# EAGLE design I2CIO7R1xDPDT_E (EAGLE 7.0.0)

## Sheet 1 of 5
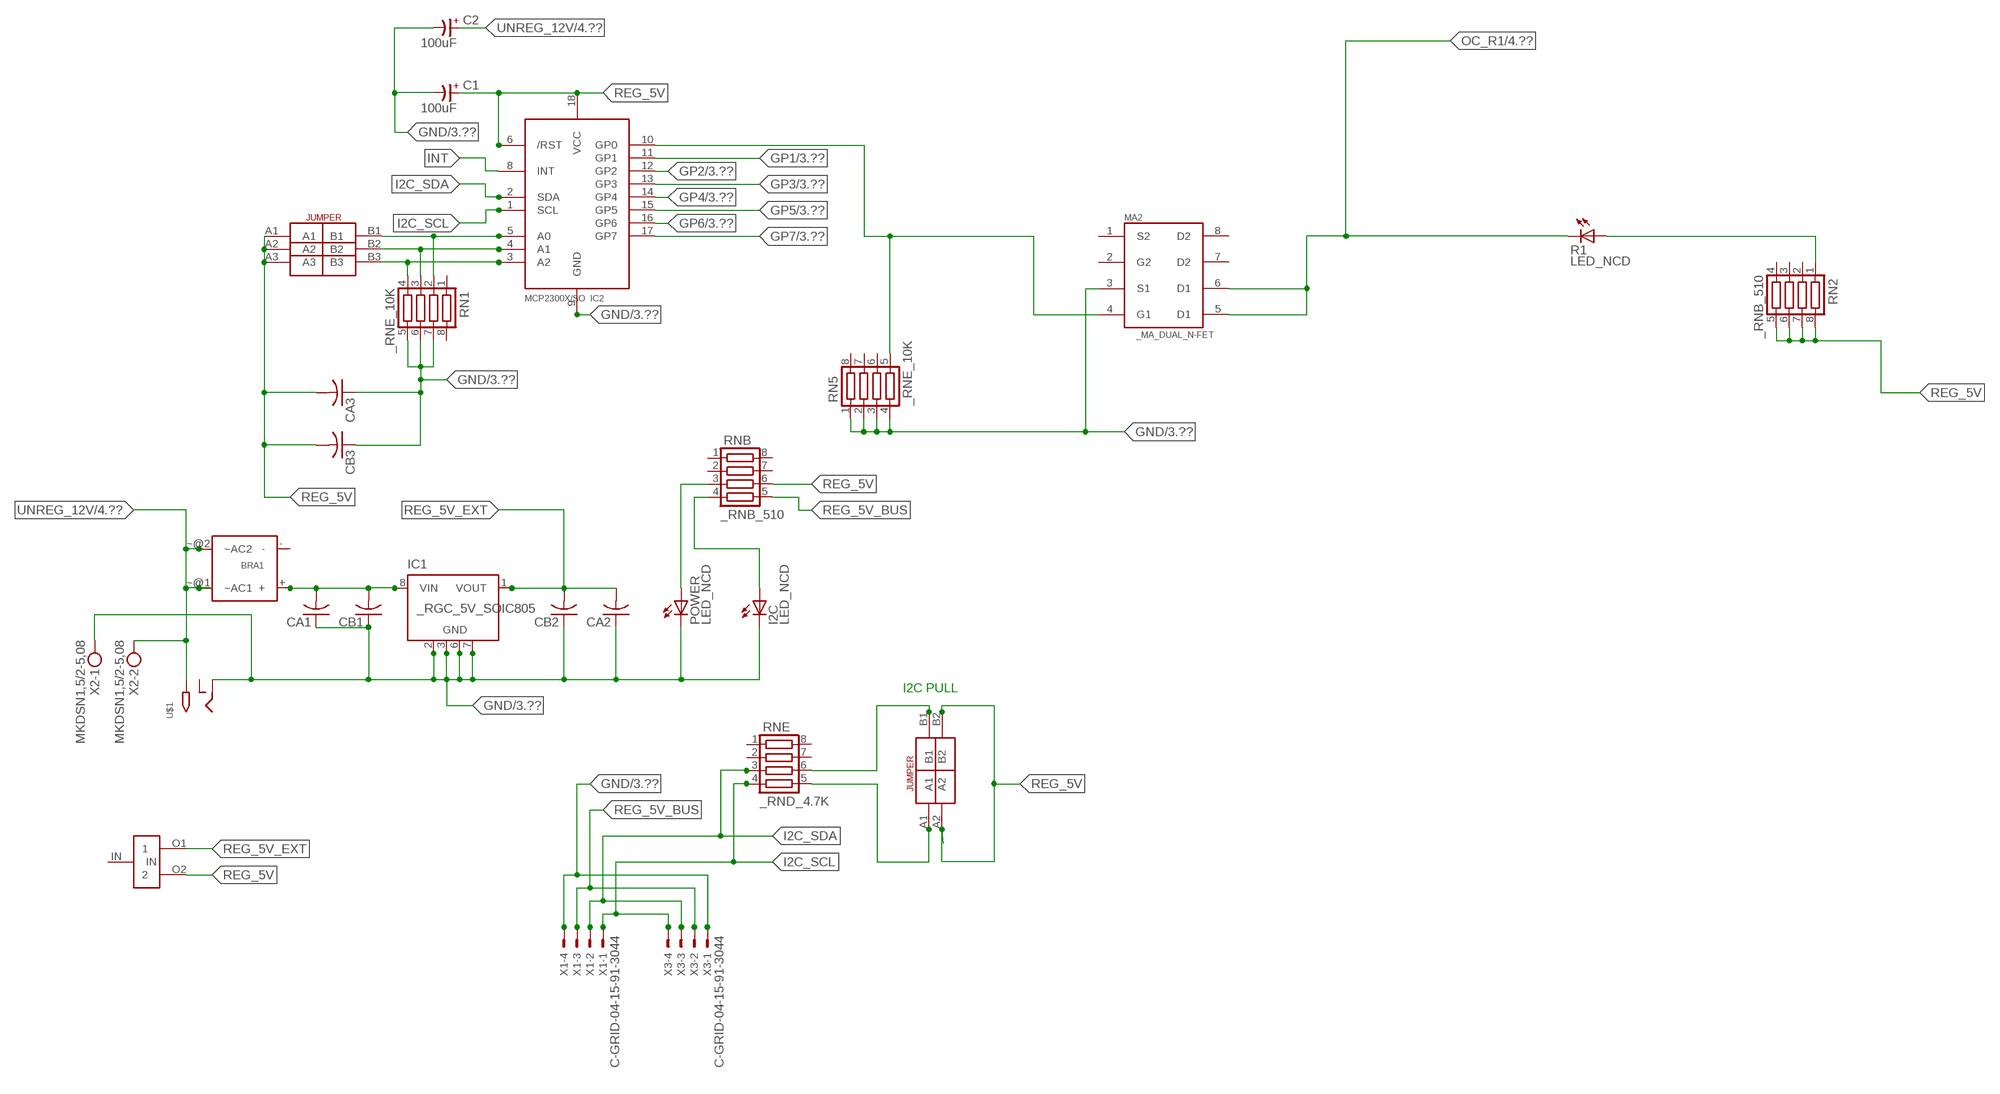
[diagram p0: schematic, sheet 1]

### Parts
BRA1  MB2S_  [MB2S]
C1  100uF  CP-E-025X060  [E-025X060]
C2  100uF  CP-E-025X060  [E-025X060]
CA1  CC1206KRX7R9BB104C1206K  [CC1206KRX7R9BB104]
CA2  CC1206KRX7R9BB104C1206K  [CC1206KRX7R9BB104]
CA3  CC1206KRX7R9BB104C1206K  [CC1206KRX7R9BB104]
CB1  TMK316F106ZL-TC1206K  [TMK316F106ZL-T]
CB2  TMK316F106ZL-TC1206K  [TMK316F106ZL-T]
CB3  TMK316F106ZL-TC1206K  [TMK316F106ZL-T]
I2C  LED_NCD  [CHIPLED_0603]
IC1  _RGC_5V_SOIC805  [_RGC_5V_SOIC8]
IC2  MCP2300X/SO  [SO18W]
MA2  _MA_DUAL_N-FET  [_MA_DUAL_N-FET]
POWER  LED_NCD  [CHIPLED_0603]
R1  LED_NCD  [CHIPLED_0603]
RN1  _RNE_10K  [RNE]
RN2  _RNB_510  [RNB]
RN5  _RNE_10K  [RNE]
RNB  _RNB_510  [RNB]
RNE  _RND_4.7K  [RND]
U$1  2.1MMJACK  [PJ-102A]
U$3  JUMPER_2X2  [JUMPER_2X2]
U$5  LINK_2  [LINK_2]
U$18  JUMPER_3X2  [JUMPER_3X2]
X1  C-GRID-04-15-91-3044  [15-91-04]
X2  MKDSN1,5/2-5,08  [MKDSN1,5/2-5,08]
X3  C-GRID-04-15-91-3044  [15-91-04]

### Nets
GND: C1.- C2.- CA1.1 CA2.1 CA3.1 CB1.1 CB2.1 CB3.1 I2C.C IC1.2(GND) IC1.3(GND) IC1.6(GND) IC1.7(GND) IC2.9(GND) MA2.3(S1) POWER.C RN1.5 RN1.6 RN1.7 RN5.1 RN5.2 RN5.3 RN5.4 U$1.RING X1.4 X2.1 X3.1 ; also sheet 3
GP1: IC2.11(GP1) ; also sheet 3
GP2: IC2.12(GP2) ; also sheet 3
GP3: IC2.13(GP3) ; also sheet 3
GP4: IC2.14(GP4) ; also sheet 3
GP5: IC2.15(GP5) ; also sheet 3
GP6: IC2.16(GP6) ; also sheet 3
GP7: IC2.17(GP7) ; also sheet 3
I2C_SCL: IC2.1(SCL) RNE.4 X1.1 X3.4
I2C_SDA: IC2.2(SDA) RNE.3 X1.2 X3.3
INT: IC2.8(INT)
N$1: BRA1.+ CA1.2 CB1.2 IC1.8(VIN)
N$2: POWER.A RNB.3
N$3: I2C.A RNB.4
N$4: RNE.5 U$3.A1
N$5: RNE.6 U$3.B1
N$6: IC2.5(A0) RN1.2 U$18.B1
N$7: IC2.4(A1) RN1.3 U$18.B2
N$8: IC2.3(A2) RN1.4 U$18.B3
N$23: IC2.10(GP0) MA2.4(G1) RN5.5
N$32: R1.A RN2.1
OC_R1: MA2.5(D1) MA2.6(D1) R1.C ; also sheet 4
REG_5V: C1.+ CA3.2 CB3.2 IC2.6(/RST) IC2.18(VCC) RN2.5 RN2.6 RN2.7 RN2.8 RNB.6 U$3.A2 U$3.B2 U$5.O2 U$18.A1 U$18.A2 U$18.A3
REG_5V_BUS: RNB.5 X1.3 X3.2
REG_5V_EXT: CA2.2 CB2.2 IC1.1(VOUT) U$5.O1
UNREG_12V: BRA1.~@1(~AC1) BRA1.~@2(~AC2) C2.+ U$1.TIP X2.2 ; also sheet 4
Unconnected: BRA1.- IC1.4(NC) IC1.5(NC) MA2.2(G2) MA2.7(D2) MA2.8(D2) RN1.1 RN1.8 RN2.2 RN2.3 RN2.4 RN5.6 RN5.7 RN5.8 RNB.1 RNB.2 RNB.7 RNB.8 RNE.1 RNE.2 RNE.7 RNE.8 U$1.RING_SW U$5.IN

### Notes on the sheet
- I2C PULL

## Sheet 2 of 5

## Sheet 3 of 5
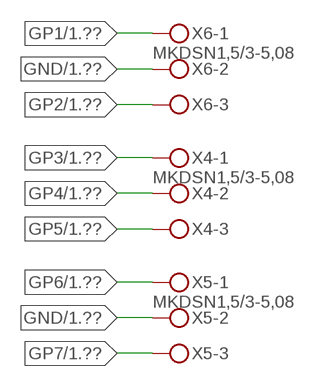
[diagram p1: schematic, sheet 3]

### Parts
X4  MKDSN1,5/3-5,08  [MKDSN1,5/3-5,08]
X5  MKDSN1,5/3-5,08  [MKDSN1,5/3-5,08]
X6  MKDSN1,5/3-5,08  [MKDSN1,5/3-5,08]

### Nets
GND: X5.2 X6.2 ; also sheet 1
GP1: X6.1 ; also sheet 1
GP2: X6.3 ; also sheet 1
GP3: X4.1 ; also sheet 1
GP4: X4.2 ; also sheet 1
GP5: X4.3 ; also sheet 1
GP6: X5.1 ; also sheet 1
GP7: X5.3 ; also sheet 1

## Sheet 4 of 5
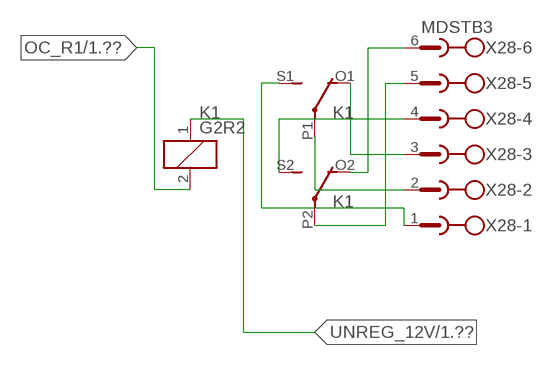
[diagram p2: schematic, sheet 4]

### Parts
K1  G2R2  [G2R2]
X28  MDSTB3  [MDSTB3]

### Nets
N$203: K1.P2(3:COM) X28.5
N$204: K1.O2(3:NC) X28.6
N$205: K1.S2(3:NO) X28.4
N$206: K1.P1(2:COM) X28.2
N$207: K1.O1(2:NC) X28.3
N$208: K1.S1(2:NO) X28.1
OC_R1: K1.2(1:C2) ; also sheet 1
UNREG_12V: K1.1(1:C1) ; also sheet 1

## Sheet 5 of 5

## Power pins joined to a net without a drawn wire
S2: MA2.1(S2)

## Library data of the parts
BRA1 = NCD_ULTIMATE_LIBRARY:MB2S: Bridge Rectifier BRA MB2S 200V 500ma Digikey MB2S-TPMSTR-ND/MB2S-TP
C1 C2 = NCD_ULTIMATE_LIBRARY:CP-: Capacitors All Kinds POLARIZED CAP
CA1-CA3 = NCD_ULTIMATE_LIBRARY:CC1206KRX7R9BB104: Capacitor CA .1uF 50V SMT C1206K CC1206KRX7R9BB104
CB1-CB3 = NCD_ULTIMATE_LIBRARY:TMK316F106ZL-T: Capacitor CB 10uF SMT 1206 TMK316F106ZL-T
I2C POWER = NCD_ULTIMATE_bhaskar:LED_NCD
IC1 = NCD_ULTIMATE_LIBRARY:_RGC_5V_SOIC8: Regulator Linear 5V Chip Positive VOLTAGE REGULATOR Digikey 497-7267-2-ND/L78L05CD13TR
IC2 = NCD_ULTIMATE_LIBRARY:MCP2300X: Semiconductor Port Expander I/O 8-Bit I2C MCP23008 Inexpensive i2c i/o expander - 8 general purpose i/o pins with optional pullups
K1 = NCD_ULTIMATE_LIBRARY:G2R2: RELAY 2 x switch, Omron
MA2 = NCD_ULTIMATE_LIBRARY:_MA_DUAL_N-FET: FET Dual N-Channel 8-SOIC NMOSFET Digikey 785-1064-2-ND/AO4842
R1 = NCD_ULTIMATE_LIBRARY:LED_NCD: LED Digikey 754-1132-2-ND/APT2012SRCPRV
RN1 RN5 = NCD_ULTIMATE_LIBRARY:_RNE_10K: Resistor Array RNE SMT 10K x 4 Single Resistor Source: http://www.ctscorp.com/components/Datasheets/CTSChipArrayDs.pdf Digikey 742C083103JPTR-ND/742C083103JP; OC_FARNELL: unknown; OC_NEWARK: unknown
RN2 RNB = NCD_ULTIMATE_LIBRARY:_RNB_510: Resistor Array RNB SMT 510 x 4 Single Resistor Source: http://www.ctscorp.com/components/Datasheets/CTSChipArrayDs.pdf Digikey 742C083511JPTR-ND/ 742C083511JP; OC_FARNELL: unknown; OC_NEWARK: unknown
RNE = NCD_ULTIMATE_LIBRARY:_RND_4.7K: Resistor Array RND SMT 4.7K x 4 Single Resistor Source: http://www.ctscorp.com/components/Datasheets/CTSChipArrayDs.pdf Digikey 742C083472JPTR-ND/742C083472JP; OC_FARNELL: unknown; OC_NEWARK: unknown
U$1 = NCD_ULTIMATE_CONNECTORS:2.1MMJACK: 2.1mm x 5.5mm DC jack with internal switch. Digikey part #PJ-102A, 4UCON part #05537 By microbuilder.eu
U$3 = NCD_ULTIMATE_CONNECTORS:JUMPER_2X2
U$5 = NCD_ULTIMATE_LIBRARY:LINK_2: PAD_top
U$18 = NCD_ULTIMATE_CONNECTORS:JUMPER_3X2
X1 X3 = NCD_ULTIMATE_CONNECTORS:C-GRID-04: CONNECTOR 4-Pos I2C wire to board 2.54 mm (0.100") pitch header Digikey WM1342-ND/0015912045; OC_FARNELL: unknown; OC_NEWARK: unknown
X2 = NCD_ULTIMATE_CONNECTORS:MKDSN1,5/2-5,08: MKDSN 1,5/ 2-5,08 Printklemme
X4-X6 = NCD_ULTIMATE_CONNECTORS:MKDSN1,5/3-5,08: MKDSN 1,5/ 3-5,08 Printklemme Nennstrom: 13,5 A Nennspannung: 250 V Rastermaß: 5,08 mm Polzahl: 3 Anschlussart: Schraubanschluss Montage: Löten Anschlussrichtung Leiter/Platine: 0 ° Artikelnummer: 1729131 Source: http://eshop.phoenixcontact.com .. 1729131.pdf
X28 = NCD_ULTIMATE_LIBRARY:MDSTB3: PHOENIX

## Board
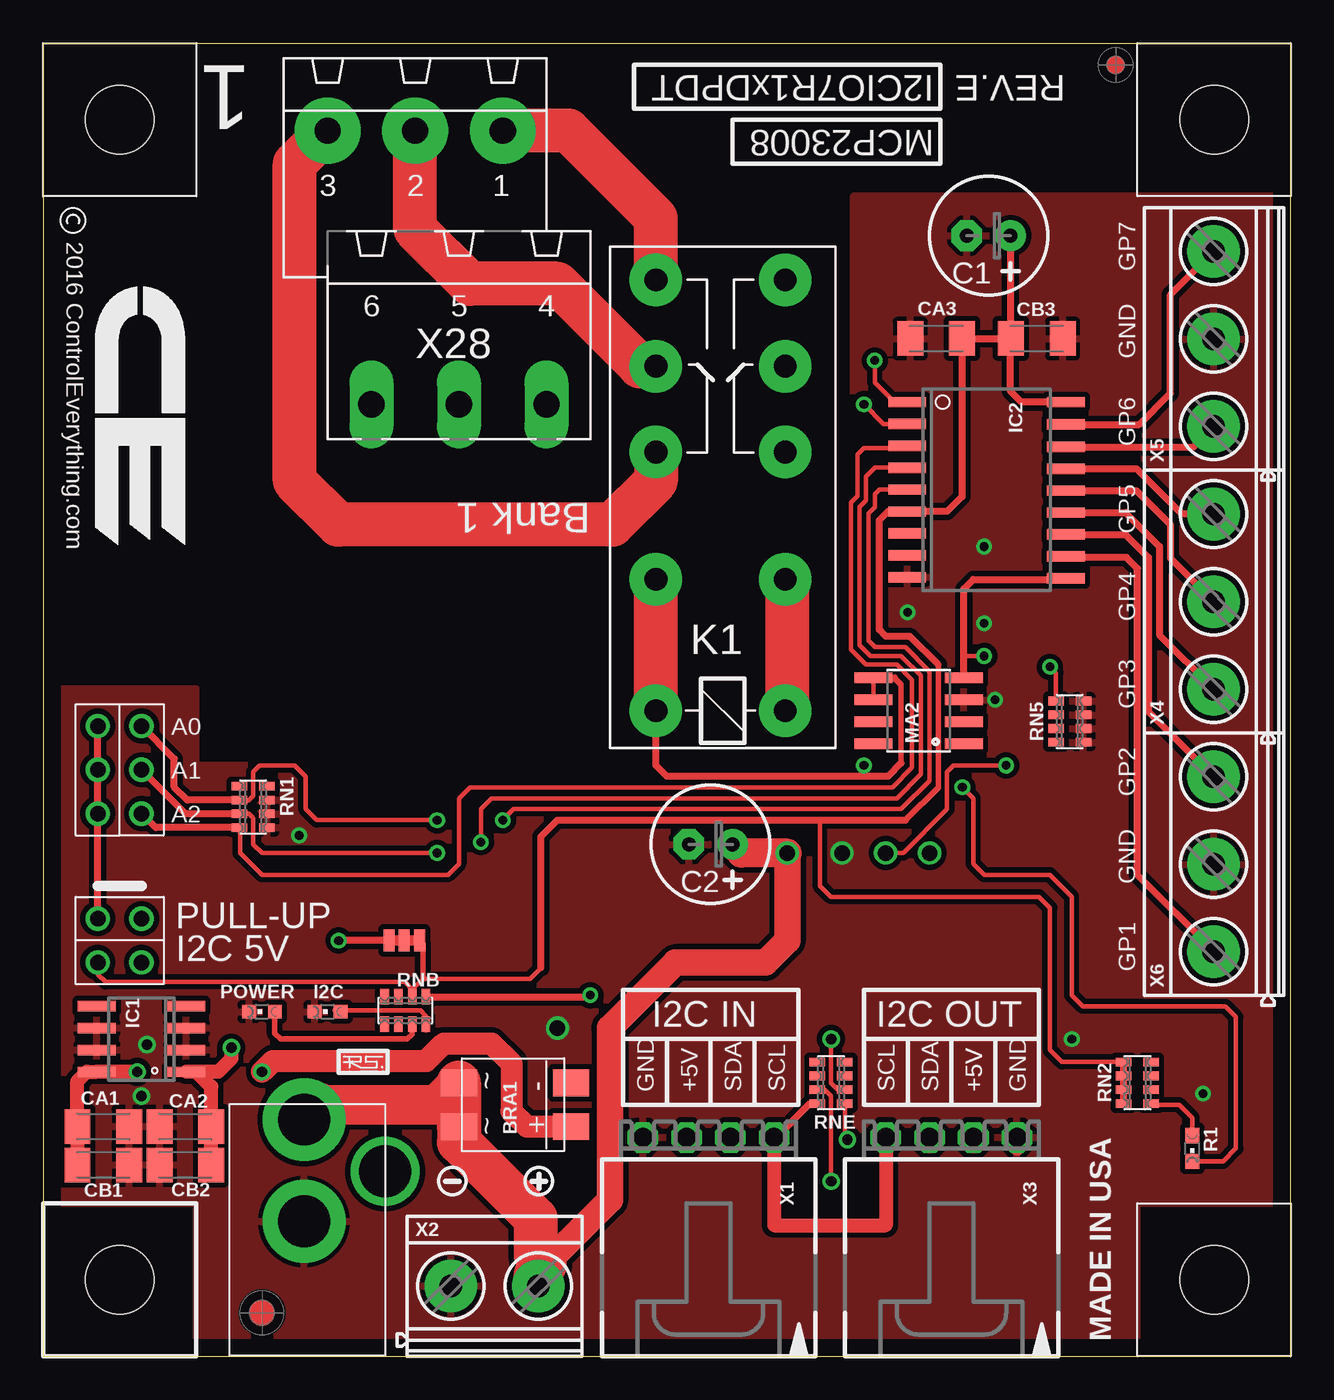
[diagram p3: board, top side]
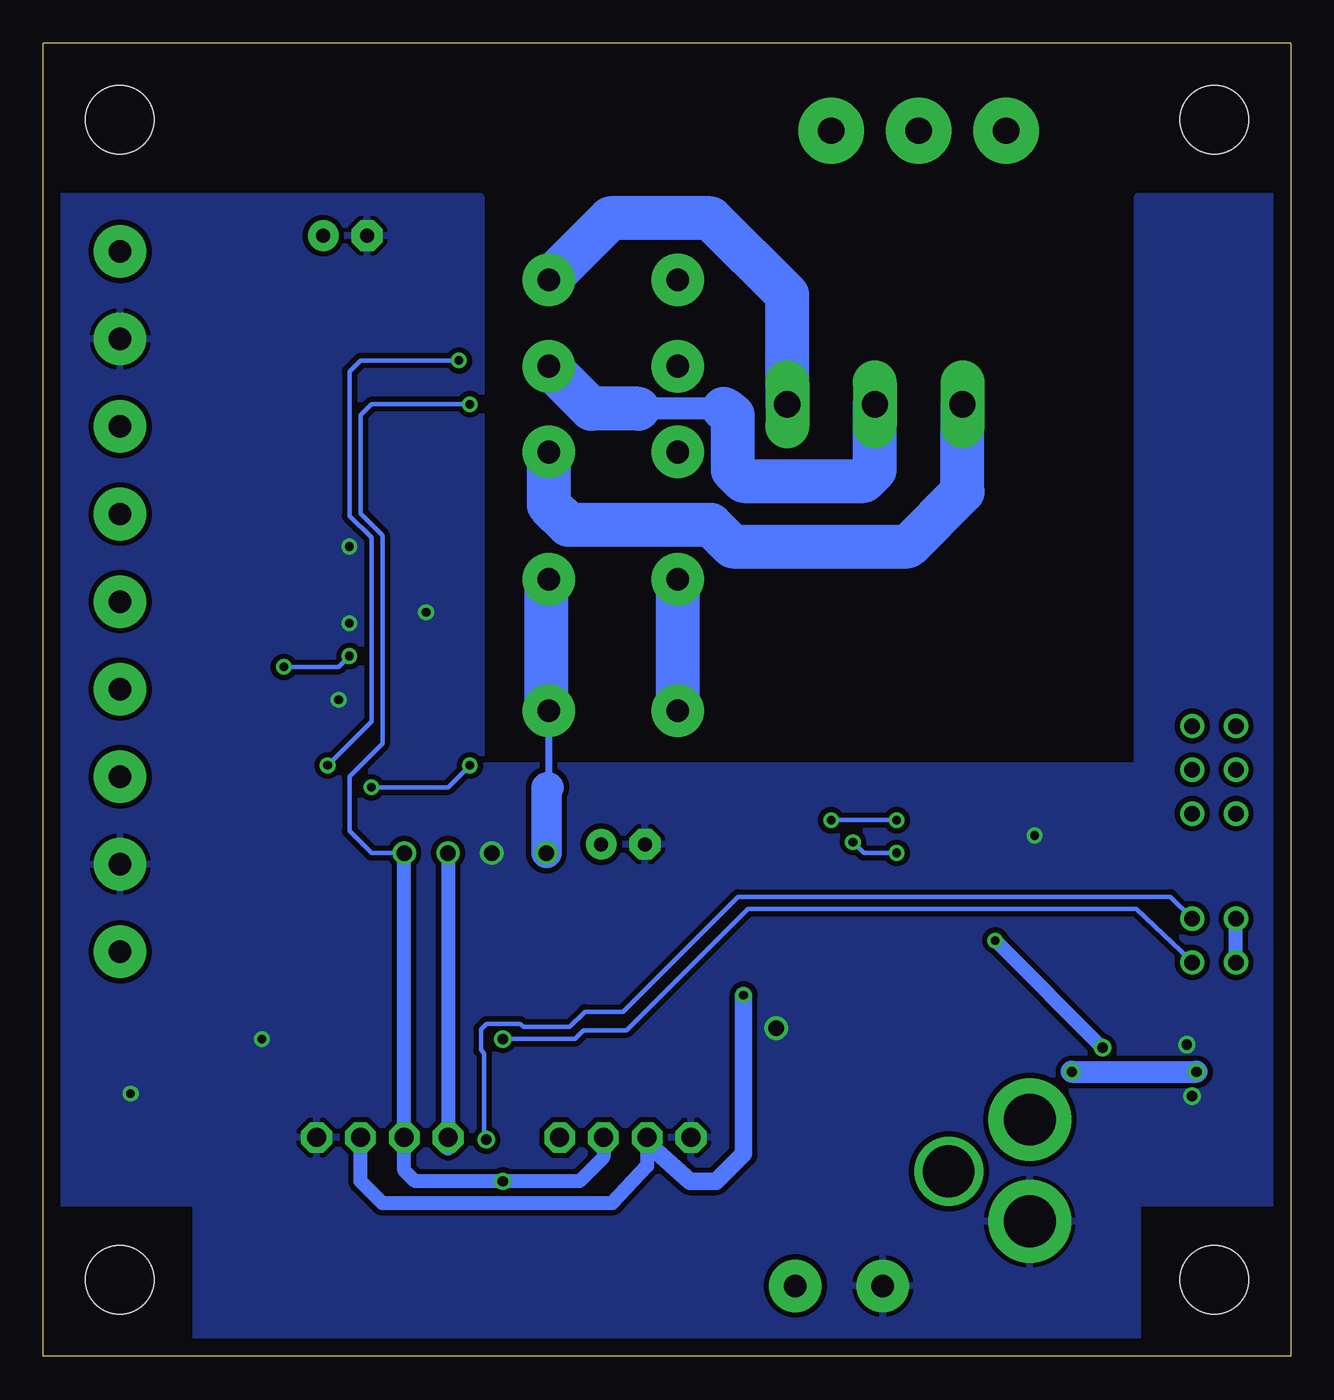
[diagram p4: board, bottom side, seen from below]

Size 72.39 x 76.2 mm. Coordinates in mm from the lower left corner, seen from the top.
Outline: 59.69,0 0,0 0,76.2 72.39,76.2 72.39,0 59.69,0
Outline: 59.69,0 61.58,0
Copper layers (1*16): Top 0.035mm / dielectric 1.5mm / Bottom 0.035mm
Design rules "default": minimum track width 10mil, minimum drill 24mil, track to track 8mil, track to pad 8mil, pad to pad 8mil, via to via 8mil, smd to smd 8mil, copper to edge 40mil, drill to drill 8mil, minimum pad ring 10mil, minimum via ring 8mil, stop-mask expansion 4mil, vias tented up to drill 0mil, thermal gap 10mil
Holes 3.96 mm at 4.45,4.45

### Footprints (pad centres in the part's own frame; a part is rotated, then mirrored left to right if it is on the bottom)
MB2S = smd 1.55 x 2.1: + 0,-6.5; - 2.54,-6.5; ~@1 0,0; ~@2 2.54,0
E-025X060 = drill 0.813 pad 1.778: + -1.27,0 | drill 0.813 pad 1.778 octagon: - 1.27,0
CC1206KRX7R9BB104 = smd 1.5 x 2: 1 -1.5,0; 2 1.5,0
TMK316F106ZL-T = smd 1.5 x 2: 1 -1.5,0; 2 1.5,0
CHIPLED_0603 = smd 0.8 x 0.8: A 0,-0.75; C 0,0.75
_RGC_5V_SOIC8 = smd 0.6 x 2.2: 1 -1.905,-2.6; 2 -0.635,-2.6; 3 0.635,-2.6; 4 1.905,-2.6; 5 1.905,2.6; 6 0.635,2.6; 7 -0.635,2.6; 8 -1.905,2.6
SO18W = smd 0.6 x 2.2: 1 -4.445,-4.6; 2 -3.175,-4.6; 3 -1.905,-4.6; 4 -0.635,-4.6; 5 0.635,-4.6; 6 1.905,-4.6; 7 3.175,-4.6; 8 4.445,-4.6; 9 5.715,-4.6; 10 5.775,4.6; 11 4.505,4.6; 12 3.235,4.6; 13 1.965,4.6; 14 0.695,4.6; 15 -0.575,4.6; 16 -1.845,4.6; 17 -3.145,4.6; 18 -4.445,4.6
G2R2 = drill 1.321 pad 3.048: 1 -2.54,-3.683; 2 -2.54,3.81; 3 5.08,-3.683; 4 5.08,3.81; O1 12.471,3.81; O2 12.471,-3.683; P1 17.45,3.81; P2 17.45,-3.683; S1 22.454,3.81; S2 22.454,-3.683
_MA_DUAL_N-FET = smd 0.61 x 2.21: 1 -1.905,-2.616; 2 -0.635,-2.616; 3 0.635,-2.616; 4 1.905,-2.616; 5 1.905,2.616; 6 0.635,2.616; 7 -0.635,2.616; 8 -1.905,2.616
CHIPLED_0603' = smd 0.8 x 0.876: A 0,-0.75; C 0,0.75
RNE = smd 0.5 x 0.9: 1 -1.2,-0.8; 2 -0.4,-0.8; 3 0.4,-0.8; 4 1.2,-0.8; 5 1.2,0.8; 6 0.4,0.8; 7 -0.4,0.8; 8 -1.2,0.8
RNB = smd 0.5 x 0.9: 1 -1.2,-0.8; 2 -0.4,-0.8; 3 0.4,-0.8; 4 1.2,-0.8; 5 1.2,0.8; 6 0.4,0.8; 7 -0.4,0.8; 8 -1.2,0.8
RND = smd 0.5 x 0.9: 1 -1.2,-0.8; 2 -0.4,-0.8; 3 0.4,-0.8; 4 1.2,-0.8; 5 1.2,0.8; 6 0.4,0.8; 7 -0.4,0.8; 8 -1.2,0.8
PJ-102A = drill 3 pad 4.8: RING 0.1,-3.39; TIP 0.1,-9.29 | drill 3 pad 3.251: RING_SW -4.6,-6.29
JUMPER_2X2 = drill 0.9: A1 0,2.54; A2 0,0; B1 2.54,2.54; B2 2.54,0
PCB_MOUNTING_HOLE = hole 3.962: 4.445,4.445
LINK_2 = smd 1.27 x 0.635: IN 0,0; O1 0,0.889; O2 0,-0.889
JUMPER_3X2 = drill 0.9: A1 0,5.08; A2 0,2.54; A3 0,0; B1 2.54,5.08; B2 2.54,2.54; B3 2.54,0
15-91-04 = drill 1.1 pad 1.778 octagon: 1 -3.81,-7.62; 2 -1.27,-7.62; 3 1.27,-7.62; 4 3.81,-7.62
MKDSN1,5/2-5,08 = drill 1.3 pad 3.048: 1 -2.561,0.025; 2 2.519,0.025
MKDSN1,5/3-5,08 = drill 1.3 pad 3.048: 1 -7.641,0.025; 2 -2.561,0.025; 3 2.519,0.025
MDSTB3 = drill 1.524 pad 3.81: 1 -3.81,-10.795; 2 1.27,-10.795; 3 6.35,-10.795 | drill 1.524 pad 2.54 long: 4 -6.35,5.08; 5 -1.27,5.08; 6 3.81,5.08

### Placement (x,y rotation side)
BRA1  24.13,13.34 90 top
C1  54.86,65.02 180 top
C2  38.73,29.72 180 top
CA1  3.49,13.34 180 top
CA2  8.26,13.34 0 top
CA3  51.82,59.05 0 top
CB1  3.49,11.11 180 top
CB2  8.26,11.11 0 top
CB3  57.66,59.05 180 top
I2C  16.51,20 90 top
IC1  5.71,18.41 90 top
IC2  54.74,50.93 270 top
K1  39.37,40.01 90 top
MA2  50.8,37.47 90 top
POWER  12.7,20 90 top
R1  LED_NCD  [CHIPLED_0603']  66.67,12.06 180 top
RN1  12.19,31.88 270 top
RN2  63.5,15.88 90 top
RN5  59.56,36.83 90 top
RNB  21.02,20.07 0 top
RNE  45.72,15.88 270 top
U$1  15.24,4.45 180 top
U$3  3.17,25.4 270 top
U$4  PCB_MOUNTING_HOLE  [PCB_MOUNTING_HOLE]  72.39,67.31 90 top
U$5  20.95,24.13 90 top
U$6  PCB_MOUNTING_HOLE  [PCB_MOUNTING_HOLE]  72.39,0 90 top
U$7  PCB_MOUNTING_HOLE  [PCB_MOUNTING_HOLE]  8.89,67.31 90 top
U$10  [VISION_REF15]  12.7,2.54 0 top
U$18  3.17,31.5 0 top
U$19  [VISION_REF10]  62.23,74.93 0 top
U$21  [ICON_USA]  61.98,0.89 90 top
U$22  [ICON_MINUS]  23.75,10.16 180 top
U$24  [ICON_PLUS]  28.77,10.16 90 top
X1  38.61,5.08 180 top
X2  26.23,4.06 0 top
X3  52.7,5.08 180 top
X4  67.94,46.35 90 top
X5  67.94,61.59 90 top
X6  67.94,31.11 90 top
X28  22.86,60.33 180 top

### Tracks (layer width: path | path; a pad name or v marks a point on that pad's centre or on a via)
GND  (via drill 0.5, 0.6, 0.9)
  Top 0.406: 34.8,12.38 X1.4
  Top 0.813: X3.1 56.52,12.06
  other vias: 5.71,15.11 6.03,18.1 46.35,29.21 29.84,19.05 14.86,30.23 54.61,42.55 54.61,46.99 59.69,18.41 67.31,15.24 50.16,43.18 55.24,38.1
  pour Bottom (isolate 0.305): -0.64,8.89 8.89,8.89 8.89,0 63.5,0 63.5,8.89 71.75,8.89 71.75,67.31 46.99,67.31 46.99,34.29 8.89,34.29 8.89,67.31 -0.64,67.31
  pour Top (isolate 0.305): -0.64,8.89 8.89,8.89 8.89,0 63.5,0 63.5,8.89 71.75,8.89 71.75,67.31 46.99,67.31 46.99,34.29 8.89,34.29 8.89,38.73 -0.64,38.73
GP1
  Top 0.406: X6.1 67.92,23.52 63.5,27.94 63.5,45.72 62.87,46.35 59.4,46.35 IC2.11
GP2
  Top 0.406: IC2.12 62.8,47.69 64.14,46.35 64.14,37.42 X6.3
GP3
  Top 0.406: IC2.13 62.8,48.96 64.77,46.99 64.77,41.86 X4.1
GP4
  Top 0.406: IC2.14 63.43,50.23 65.41,48.26 65.41,46.31 X4.2
GP5
  Top 0.406: IC2.15 63.43,51.5 66.04,48.9 67.9,48.9 X4.3
GP6
  Top 0.406: IC2.16 66.74,52.77 X5.1
GP7
  Top 0.406: IC2.17 63.6,54.07 65.41,55.88 65.41,61.6 X5.3
I2C_SCL  (via drill 0.5, 0.9)
  Top 0.254: IC2.1 49.4,55.37 48.26,56.52 v48.26,57.78 | v55.88,34.29 52.83,34.29 52.45,33.91 52.45,31.75 49.91,29.21 v48.9,29.21
  Top 0.406: RNE.4 44.51,14.68 42.42,12.57
  Top 0.813: X3.4 48.9,7.62 42.42,7.62 42.42,12.57 X1.1
  Bottom 0.254: v48.26,57.78 53.98,57.78 54.61,57.15 54.61,48.77 53.34,47.5 53.34,36.83 v55.88,34.29
  Bottom 0.813: v48.9,29.21 X3.4 48.9,12.06
I2C_SDA  (via drill 0.5, 0.6, 0.9)
  Top 0.254: RNE.3 45.36,15.47 45.72,15.11 v45.72,10.16 | IC2.2 48.77,54.1 v47.62,55.24
  Top 0.61: X3.3 51.44,12.06 | X1.2 39.88,12.38
  Bottom 0.254: v47.62,55.24 53.34,55.24 53.98,54.61 53.98,48.9 52.7,47.62 52.7,35.56 54.61,33.66 54.61,30.48 53.34,29.21 v51.44,29.21
  Bottom 0.406: 39.88,12.38 X1.2
  Bottom 0.813: 39.88,12.38 39.88,11.56 41.27,10.16 v45.72,10.16 50.8,10.16 51.44,10.79 X3.3 v51.44,29.21
N$1  (via drill 0.6)
  Top 0.813: CB1.2 CA1.2 1.99,15.96 2.54,16.51 IC1.8 v5.46,16.51
  Top 1.27: v12.7,16.51 13.34,17.14 22.23,17.14 23.24,18.16 26.04,18.16 27.18,17.02 27.18,14.22 28.07,13.34 BRA1.+
  Bottom 1.27: v12.7,16.51 v5.46,16.51
N$2
  Top 0.305: RNB.3 21.4,18.95 21.4,18.7 21.12,18.41 13.78,18.41 13.45,18.74 POWER.A
N$3
  Top 0.254: 22.23,18.95 22.23,19.74 21.9,20.07 16.94,20.07
  Top 0.305: RNB.4 22.23,18.95 | 16.94,20.07 I2C.A
N$4  (via drill 0.6)
  Top 0.254: RNE.5 46.52,12.6 v46.67,12.57
  Bottom 0.254: U$3.A1 6.99,26.67 32.07,26.67 38.73,20 40.96,20 41.85,19.11 44.51,19.11 44.7,19.3 46.67,19.3 46.99,18.99 46.99,17.78 46.8,17.59 46.8,12.7 v46.67,12.57
N$5  (via drill 0.6)
  Top 0.254: RNE.6 46.12,15.47 45.72,15.88 v45.72,18.41
  Bottom 0.254: v45.72,18.41 41.53,18.41 41.02,18.92 38.54,18.92 31.5,25.97 8.95,25.97 6.35,23.5 U$3.B1
N$6  (via drill 0.5)
  Top 0.254: v26.67,31.11 27.3,31.75 49.78,31.75 51.44,33.4 51.44,39.75 50.04,41.15 48.26,41.15 47.88,41.53 47.88,48.9 48.26,49.28 48.26,50.04 48.51,50.29 IC2.5 50.01,50.16 | v22.86,31.11 15.88,31.11 15.24,31.75 15.24,33.66 14.61,34.29 12.57,34.29 12.19,33.91 12.19,32.51 11.94,32.26 11.41,32.26 RN1.2
  Top 0.406: RN1.2 8.36,32.28 7.62,33.02 7.62,34.67 U$18.B1
  Bottom 0.254: v26.67,31.11 v22.86,31.11
N$7  (via drill 0.5)
  Top 0.254: v25.4,29.84 25.4,31.75 26.04,32.38 49.53,32.38 50.93,33.78 50.93,39.5 49.78,40.64 48.01,40.64 47.37,41.27 47.37,49.28 47.75,49.66 47.75,51.05 48.26,51.56 IC2.4 50.01,51.44 | v22.86,29.21 12.7,29.21 12.19,29.72 12.19,31.24 11.94,31.5 11.41,31.5 RN1.3
  Top 0.406: RN1.3 8.27,31.48 U$18.B2
  Bottom 0.254: v25.4,29.84 24.77,29.21 v22.86,29.21
N$8
  Top 0.254: RN1.4 11.43,30.64 11.43,29.21 12.7,27.94 23.5,27.94 24.13,28.57 24.13,32.38 24.77,33.02 49.28,33.02 50.42,34.16 50.42,39.24 49.53,40.13 47.75,40.13 46.86,41.02 46.86,49.53 47.24,49.91 47.24,52.32 47.62,52.7 50.01,52.7 IC2.3
  Top 0.406: RN1.4 6.53,30.68 U$18.B3
N$23  (via drill 0.5)
  Top 0.254: RN5.5 58.76,39.66 v58.42,40.01 | v54.61,40.64 53.42,40.64
  Top 0.406: MA2.4 53.42,40.64 53.42,44.53 53.98,45.09 59.27,45.09 IC2.10
  Bottom 0.254: v58.42,40.01 55.24,40.01 v54.61,40.64
N$32
  Top 0.254: R1.A 66.67,13.84 65.91,14.61 64.37,14.61 RN2.1
N$203
  Bottom 1.27: 32.89,54.99 37.85,54.99
  Bottom 2.54: 24.13,53.98 X28.5 24.13,51.44 24.77,50.8 31.75,50.8 32.38,51.44 32.38,54.61 32.89,54.99 | 37.85,54.99 40.59,54.99 K1.P2
N$204
  Bottom 2.54: K1.O2 43.05,49.4 41.91,48.26 33.66,48.26 32.38,46.99 22.23,46.99 19.05,50.16 X28.6
N$205
  Bottom 2.54: X28.4 29.21,61.59 33.66,66.04 39.47,66.04 K1.S2
N$206
  Top 2.54: K1.P1 34.62,57.45 29.84,62.23 24.77,62.23 21.59,65.41 X28.2
N$207
  Top 2.54: K1.O1 35.56,50.8 33.02,48.26 17.14,48.26 14.61,50.8 14.61,69.22 X28.3
N$208
  Top 2.54: K1.S1 35.56,66.04 30.48,71.12 X28.1
OC_R1  (via drill 0.5)
  Top 0.254: MA2.5 MA2.6 | R1.C 68.47,11.31 69.22,12.06 69.22,19.68 68.58,20.32 60.33,20.32 59.69,20.95 59.69,26.67 58.42,27.94 54.61,27.94 53.98,28.57 53.98,32.38 v53.34,33.02 | v47.62,34.29 47.62,33.66
  Top 0.305: 49.4,39.37 49.78,38.99 49.78,34.42
  Top 0.406: MA2.5 49.4,39.37 | 49.78,34.42 49.02,33.66 47.62,33.66 36.2,33.66 35.56,34.29 K1.2
  Bottom 0.254: v53.34,33.02 48.9,33.02 v47.62,34.29
REG_5V
  Top 0.254: RNB.6 21.42,21.29 | 21.42,21.29 22.04,21.91 28.26,21.91 28.89,22.54 | 21.42,21.29 20.99,21.72 3.62,21.72 3.17,22.16 U$3.B2 | RN2.5 59.12,17.07 58.42,17.78 58.42,26.04 57.78,26.67 45.72,26.67 45.09,27.3 45.09,31.11
  Top 0.305: 50.04,31.11 51.94,33.02 51.94,40.13 | 22.04,21.91 22.04,23.94 U$5.O2
  Top 0.406: U$18.A1 U$18.A2 U$18.A3 U$3.A2 | RN2.8 RN2.7 RN2.6 RN2.5 | 28.89,22.54 28.89,30.16 29.84,31.11 45.09,31.11 50.04,31.11 | 51.94,40.13 50.29,41.78 48.9,41.78 48.51,42.16 48.51,48.51 49.02,49.02 IC2.6 52.45,49.02 53.32,49.89 CA3.2 CB3.2 56.13,59.03 | IC2.18 56.77,55.37 56.13,56.01 56.13,59.03 | C1.+ 56.13,59.03
  Bottom 0.813: U$3.B2 U$3.A2
REG_5V_BUS  (via drill 0.5)
  Top 0.406: RNB.5 31.66,20.87 v31.75,20.95
  Top 0.61: X1.3 37.34,12.38 | X3.2 53.98,12.06
  Bottom 0.406: 37.34,12.38 X1.3 | 53.98,12.06 X3.2
  Bottom 0.813: 37.34,12.38 37.34,11.05 39.37,8.89 52.7,8.89 53.98,10.16 53.98,12.06
  Bottom 1.016: 37.34,12.38 34.86,10.16 33.34,10.16 31.75,11.75 v31.75,20.95
REG_5V_EXT  (via drill 0.5, 0.6)
  Top 0.406: U$5.O1 v17.14,24.13
  Top 0.813: CB2.2 CA2.2 9.76,15.64 8.89,16.51 | 8.89,16.51 IC1.1 | v10.92,17.91 10.92,17.27 10.16,16.51 8.89,16.51
  Bottom 0.813: v17.14,24.13 v10.92,17.91
UNREG_12V  (via drill 0.9)
  Top 1.524: v43.18,29.21 43.18,24.13 41.91,22.86 36.7,22.86 32.89,19.05 32.89,9.08 29.11,5.3 28.57,4.76
  Top 1.676: v43.18,29.21 40.51,29.21 C2.+
  Top 2.286: BRA1.~@2 22.86,14.61 16.01,14.61
  Top 2.54: 16.01,14.61 U$1.TIP | X2.2 28.55,4.45 28.57,4.76 | BRA1.~@2 BRA1.~@1 24.13,12.45 28.57,8 28.57,5.84 29.11,5.3
  Bottom 0.406: 43.05,33.15 43.18,33.02 | K1.1 43.05,33.02
  Bottom 1.778: v43.18,29.21 43.18,33.02 43.05,33.02

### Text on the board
tNames: 1 | I2CIO7R1xDPDT | REV.E | MCP23008 | 2016 ControlEverything.com | GP7 | GND | GP6 | Bank 1 | GP5 | GP4 | GP3 | A0 | A1 | GP2 | A2 | GND | PULL-UP | I2C 5V | GP1 | I2C IN | I2C OUT | GND | +5V | SDA | SCL | SCL | SDA | +5V | +5V | GND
